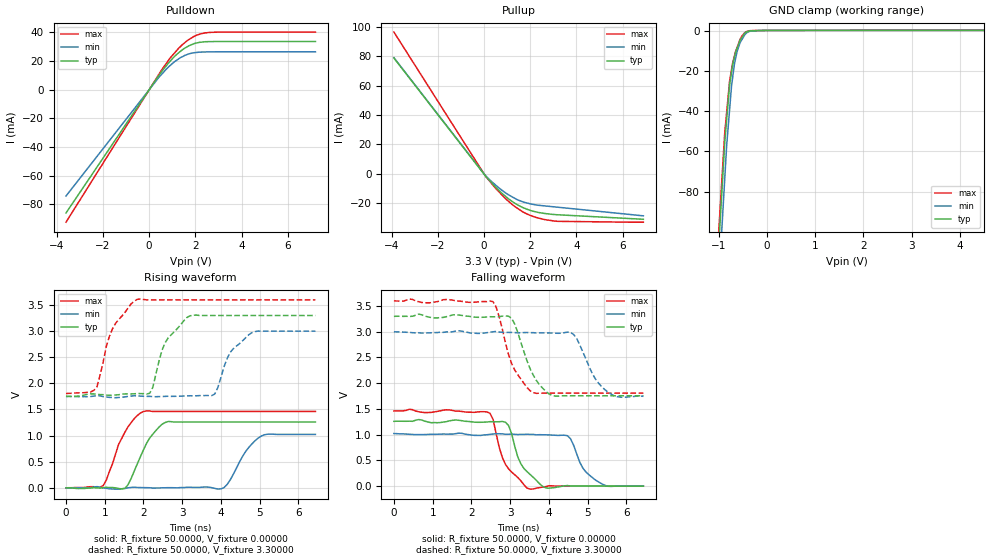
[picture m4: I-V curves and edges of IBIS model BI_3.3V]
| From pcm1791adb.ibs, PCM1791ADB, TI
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[Model] BI_3.3V
Model_type I/O
Vinl  = 800.000mV
Vinh  = 2.00000V
Vref  = 0.00000V
Cref  = 2.00000pF
Vmeas = 1.65000V
C_comp  2.00000pF 2.00000pF 2.00000pF
| variable   typ   min   max
[Voltage Range]   3.30000V  3.00000V  3.60000V
[POWER Clamp Reference]  3.30000V  3.00000V  3.60000V
[Pullup Reference]   3.30000V  3.00000V  3.60000V
[Pulldown Reference]   0.00000V  0.00000V  0.00000V
[GND Clamp Reference]   0.00000V  0.00000V  0.00000V
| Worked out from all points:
|   slope of the pulldown table from 0 to 0.495 V, typ, clamps not added: 42.7 ohm
|   slope of the pullup table from 0 to 0.495 V, typ, clamps not added: 56.2 ohm
|   GND clamp passes 1 mA (typ) near -0.45 V on its own axis
|   rising waveform, R_fixture 50.0000, V_fixture 0.00000: 20-80 % time 496ps typ, 493ps min, 492ps max; typ from 0 V to 1.26 V
|   falling waveform, R_fixture 50.0000, V_fixture 0.00000: 20-80 % time 435ps typ, 434ps min, 417ps max; typ from 1.26 V to 0 V
|   falling waveform, R_fixture 50.0000, V_fixture 3.30000: 20-80 % time 473ps typ, 494ps min, 463ps max; typ from 3.3 V to 1.75 V
|   rising waveform, R_fixture 50.0000, V_fixture 3.30000: 20-80 % time 511ps typ, 508ps min, 501ps max; typ from 1.75 V to 3.3 V
[GND Clamp]
-3.3V     -1.046A    -1.078A    -999.8mA
-881mV    -55.89mA   -73.94mA   -51.06mA
-840.9mV  -44.51mA   -57.27mA   -40.77mA
-780.3mV  -27.35mA   -39.56mA   -25.27mA
-739.7mV  -20.7mA    -27.67mA   -19.41mA
-719.4mV  -17.38mA   -23.97mA   -16.48mA
-679.1mV  -13.22mA   -16.6mA    -12.61mA
-623.4mV  -8.829mA   -10.38mA   -8.374mA
-562.1mV  -4.848mA   -6.036mA   -4.405mA
-420.8mV  -625.3uA   -1.071mA   -442.3uA
61.63mV   65.1uA     47.55uA    79.25uA
6.6V      102.1uA    79.84uA    108.8uA
[Pulldown]
-3.6V     -86.06mA   -74.22mA   -92.47mA
420.6mV   9.885mA    8.601mA    10.69mA
759.5mV   17.05mA    14.64mA    18.71mA
1.042V    22.25mA    18.76mA    24.58mA
1.361V    26.87mA    22.45mA    30.24mA
1.659V    30.06mA    24.63mA    34.36mA
2.079V    32.7mA     26.03mA    38.18mA
2.579V    33.55mA    26.38mA    39.95mA
7.2V      33.64mA    26.45mA    40.2mA
[Pullup]
-3.9V     78.78mA    78.99mA    96.47mA
77.7mV    -1.836mA   -1.578mA   -1.922mA
497.8mV   -9.11mA    -7.686mA   -9.876mA
761.3mV   -13.14mA   -11.1mA    -14.23mA
1.281V    -19.61mA   -16.35mA   -21.78mA
1.661V    -22.95mA   -19.07mA   -25.85mA
1.979V    -24.84mA   -20.44mA   -28.27mA
2.358V    -26.44mA   -21.53mA   -30.25mA
3V        -27.77mA   -22.54mA   -32.2mA
6.9V      -31.07mA   -28.73mA   -33.06mA
[POWER Clamp]
| Voltage   I(typ)   I(min)   I(max)
-3.6V     0A         0A         0A
-3.5V     0A         0A         0A
-3.4V     0A         0A         0A
7.2V      0A         0A         0A
[Rising Waveform]
R_fixture = 50.0000
V_fixture = 0.00000
V_fixture_min = 0.00000
V_fixture_max = 0.00000
0s        0V         0V         0V
960ps     3.003mV    -3.257mV   42.47mV
1.52ns    -10.73mV   -13.69mV   1.064V
2ns       726.5mV    2.48mV     1.461V
2.56ns    1.251V     179.7uV    1.462V
4ns       1.259V     -20.58mV   1.462V
4.24ns    1.259V     151.6mV    1.462V
4.64ns    1.259V     697.4mV    1.462V
5.04ns    1.259V     990mV      1.462V
6.44ns    1.259V     1.022V     1.462V
[Falling Waveform]
R_fixture = 50.0000
V_fixture = 0.00000
V_fixture_min = 0.00000
V_fixture_max = 0.00000
0s        1.259V     1.022V     1.462V
2.48ns    1.252V     1.005V     1.415V
2.88ns    1.241V     1.007V     422.1mV
3.28ns    428.6mV    1.004V     98.35mV
3.52ns    222.7mV    1.003V     -60.69mV
3.92ns    -35.94mV   996.6mV    -10.98mV
4.48ns    9.761mV    978.7mV    0V
4.88ns    0V         347mV      0V
5.44ns    0V         16.16mV    0V
6.44ns    0V         0V         0V
[Falling Waveform]
R_fixture = 50.0000
V_fixture = 3.30000
V_fixture_min = 3.00000
V_fixture_max = 3.60000
0s        3.3V       3V         3.6V
2.56ns    3.291V     2.999V     3.584V
2.96ns    3.302V     2.987V     2.555V
3.12ns    3.149V     2.984V     2.254V
3.44ns    2.427V     2.986V     1.913V
3.76ns    1.969V     2.978V     1.806V
4.08ns    1.764V     2.975V     1.806V
4.56ns    1.755V     2.987V     1.806V
5.44ns    1.755V     1.879V     1.806V
6.44ns    1.755V     1.745V     1.806V
[Rising Waveform]
R_fixture = 50.0000
V_fixture = 3.30000
V_fixture_min = 3.00000
V_fixture_max = 3.60000
0s        1.755V     1.745V     1.806V
800ps     1.791V     1.767V     1.936V
1.2ns     1.772V     1.73V      3.044V
1.84ns    1.806V     1.761V     3.61V
2.16ns    1.81V      1.751V     3.6V
2.56ns    2.779V     1.751V     3.6V
3.2ns     3.294V     1.763V     3.6V
3.84ns    3.3V       1.796V     3.6V
4.8ns     3.3V       2.972V     3.6V
6.44ns    3.3V       3V         3.6V
[Ramp]
| variable  typ   min   max
dV/dt_r   755.492m/326.348p  612.017m/326.268p  874.812m/307.716p
dV/dt_f   929.998m/347.202p  754.362m/388.409p  1.07646/335.384p
R_load = 50.0000Ohms
